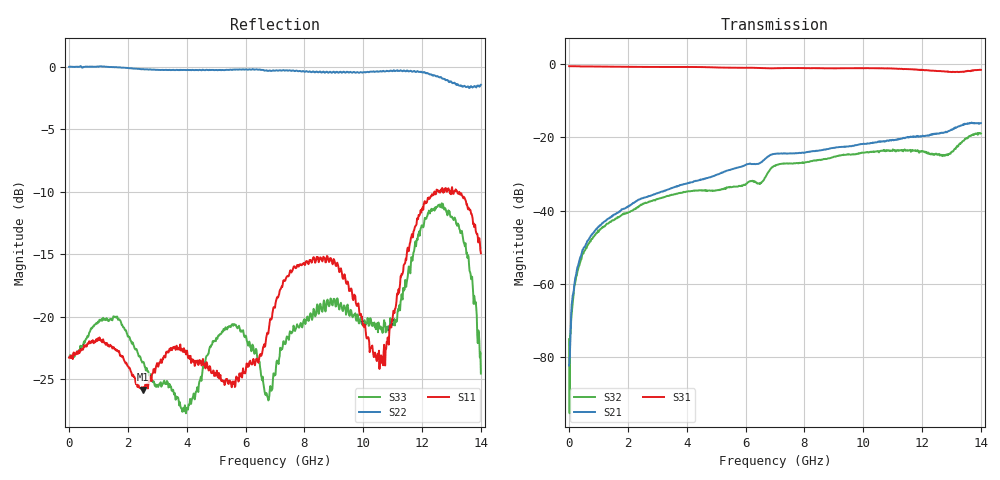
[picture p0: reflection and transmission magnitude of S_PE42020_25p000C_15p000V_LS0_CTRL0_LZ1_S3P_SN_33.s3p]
! Device ID: PE42020
! File Path: z:\PE42020\sparam_retest1\25p000C\3p000\LS_CTRL0_LZ1\PE42020_25p000C_3p000V_3p000V_0p000V_LS_CTRL0_LZ1_S3P_SN_33__2_3.s3p
! Serial: 33
! Lot:
! Temp: 25.000C
! VDD: 15.000
! VSS: -15.000
! Control_Hi: 3.000
! Control_Lo: 0.000
! Logic State: LS_CTRL0_LZ1
! Port 1: RFC
! Port 3: RF2
! Port 4:
! ThroughPath:1-4
! IDD: -0.0020383109
! ISS: 0
! Comment:
#  Hz  S  RI  R  50
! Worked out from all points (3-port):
!   801 points, 300 kHz to 14 GHz, reference 50 ohm
!   strongest paths, dB at 300 kHz, 3.5 GHz, 7 GHz, 10.5 GHz, 14 GHz:
!     S31: -0.6, -0.8, -1.1, -1.1, -1.6
!     S21: -82.2, -33.8, -24.5, -21.2, -16.1
!     S32: -75.0, -35.7, -27.8, -23.8, -19.0
!   lowest |S11| = -25.9 dB at 2.503 GHz (marker M1), VSWR 1.11, Z = 54.3 - j3.14 ohm
!   |S11| at or under -10 dB: start of sweep to 12.42 GHz; 12.42868 GHz to 12.48621 GHz (57.53 MHz wide, 0.462 % of centre); 13.2 GHz to end of sweep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
300000  0.0682 0.00519  0.000377 -0.000243  0.9348 0.000898
        6.53e-05 -4.16e-05  1.002 0.00395  2.85e-05 -8.82e-05
        0.9346 0.000229  -0.000138 0.000112  0.0685 0.00341
1.753e8  0.0685 -0.0139  -7.05e-05 0.000968  0.928 -0.0441
         -8.47e-05 0.000958  0.9987 -0.0537  -1.26e-05 0.000884
         0.9286 -0.0449  -6.04e-05 0.000929  0.0678 -0.0121
5.078e8  0.0682 -0.0351  0.000152 0.00305  0.9178 -0.122
         0.000207 0.00317  0.9898 -0.1526  0.000306 0.00278
         0.9182 -0.1223  0.000409 0.00276  0.0709 -0.0359
2.5028e9  0.042 -0.0289  0.00617 0.0135  0.7356 -0.5416
          0.00618 0.0134  0.812 -0.5492  0.00804 0.00928
          0.7351 -0.5405  0.0081 0.00929  0.0504 -0.0422
7.0003e9  0.0622 -0.0889  0.0554 0.0216  -0.1612 -0.8629
          0.0557 0.0215  -0.037 -0.9655  0.0411 0.0033
          -0.1595 -0.8616  0.0407 0.00317  0.0404 -0.042
8.9428e9  0.1017 -0.1303  0.0708 -0.01  -0.5532 -0.678
          0.0708 -0.00936  -0.4544 -0.8339  0.04 -0.0346
          -0.547 -0.6812  0.0402 -0.0348  0.0542 -0.0973
1.06228e10  0.0148 -0.0654  0.0753 -0.0448  -0.7957 -0.3735
            0.0755 -0.0458  -0.8048 -0.5222  0.0143 -0.0636
            -0.792 -0.377  0.0147 -0.0642  -0.061 -0.0635
1.26003e10  -0.0361 -0.3173  0.0627 -0.0967  -0.7964 0.0577
            0.0604 -0.0953  -0.8478 -0.3263  -0.0139 -0.0573
            -0.7996 0.0523  -0.0139 -0.0549  0.0206 -0.2801
1.34228e10  0.0536 -0.297  0.0497 -0.143  -0.7766 0.1648
            0.0493 -0.1402  -0.8387 0.014  -0.0144 -0.091
            -0.7653 0.1499  -0.014 -0.0891  0.0261 -0.1956
1.40003e10  0.0804 -0.1602  -0.00186 -0.1534  -0.7816 0.2876
            -0.000622 -0.1563  -0.7862 0.3202  -0.0601 -0.0964
            -0.7862 0.274  -0.059 -0.0962  -0.0226 -0.0546
